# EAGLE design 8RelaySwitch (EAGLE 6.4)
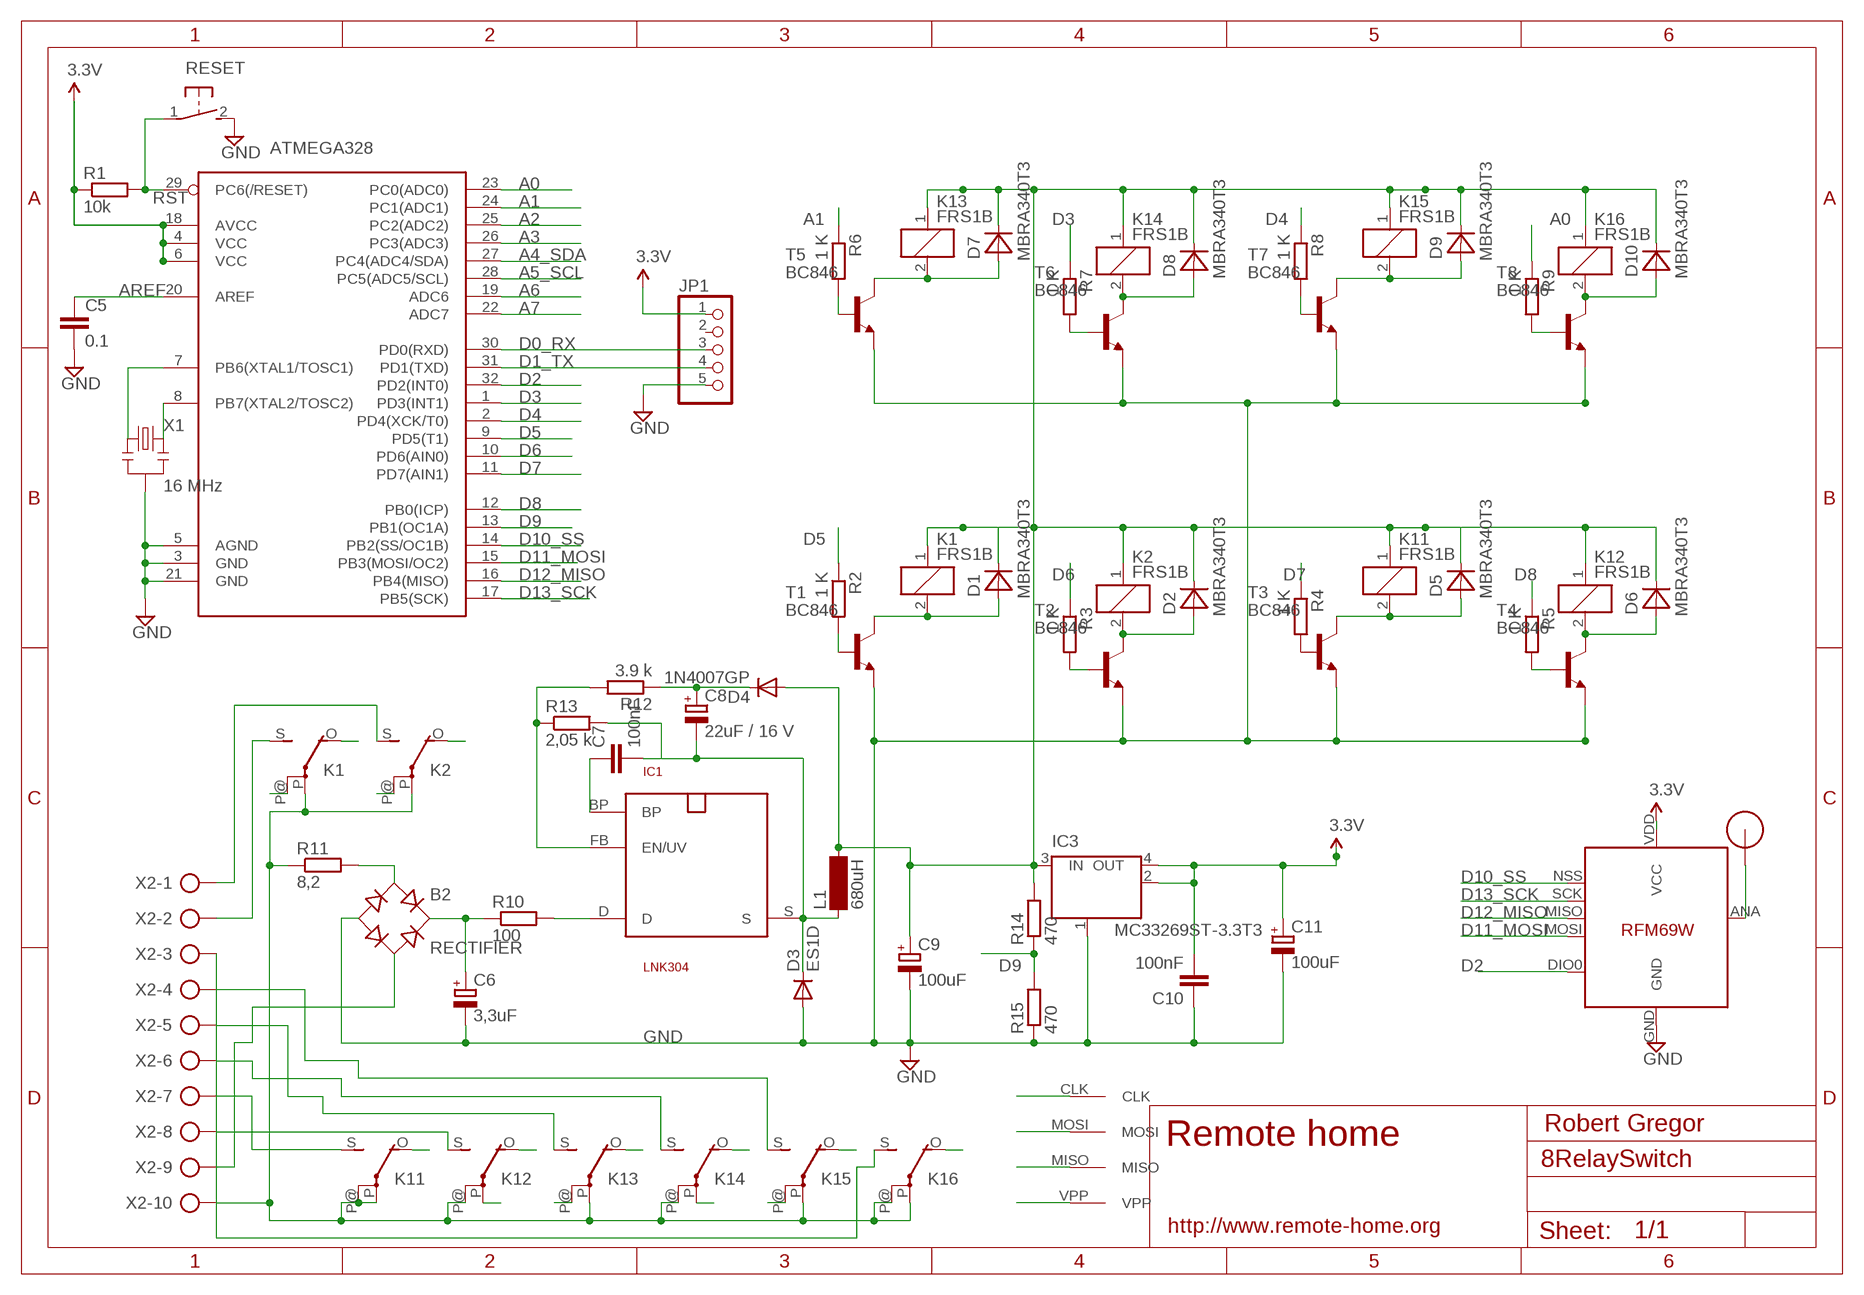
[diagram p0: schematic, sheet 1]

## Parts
ATMEGA328  ATMega-328  ATMEGA168/328TQFP32  [TQFP32-08]
B2  RECTIFIER  RECTIFIER-S40  [TO-269AA]
C5  0.1  C-EUC2012  [C2012]
C6  3,3uF  CPOL-EUE5-10.5  [E5-10,5]
C7  100nF  C-EUC2012  [C2012]
C8  22uF / 16 V  CPOL-EUSMCC  [SMC_C]
C9  100uF  CPOL-EUSMCB  [SMC_B]
C10  100nF  C-EUC2012  [C2012]
C11  100uF  CPOL-EUSMCB  [SMC_B]
D1  MBRA340T3  [SMA]
D2  MBRA340T3  [SMA]
D3  ES1D  DIODE-DO214AC  [DO214AC]
D4  1N4007GP  DIODE-DO214AA  [DO214AA]
D5  MBRA340T3  [SMA]
D6  MBRA340T3  [SMA]
D7  MBRA340T3  [SMA]
D8  MBRA340T3  [SMA]
D9  MBRA340T3  [SMA]
D10  MBRA340T3  [SMA]
IC1  LNK304  SO-8C  [SO-8C]
IC3  MC33269ST-3.3T3  [SOT223]
JP1  PINHD-1X05_2.54-S  [1X05-S]
K1  FRS1B  [FRS1B]
K2  FRS1B  [FRS1B]
K11  FRS1B  [FRS1B]
K12  FRS1B  [FRS1B]
K13  FRS1B  [FRS1B]
K14  FRS1B  [FRS1B]
K15  FRS1B  [FRS1B]
K16  FRS1B  [FRS1B]
L1  680uH  BS11  [BS11]
R1  10k  R-EU_R2012  [R2012]
R2  1 K  R-EU_M2012  [M2012]
R3  1 K  R-EU_M2012  [M2012]
R4  1 K  R-EU_M2012  [M2012]
R5  1 K  R-EU_M2012  [M2012]
R6  1 K  R-EU_M2012  [M2012]
R7  1 K  R-EU_M2012  [M2012]
R8  1 K  R-EU_M2012  [M2012]
R9  1 K  R-EU_M2012  [M2012]
R10  100  R-EU_R2512W  [R2512W]
R11  8,2  R-EU_0411/12  [0411/12]
R12  3.9 k  R-EU_M2012  [M2012]
R13  2,05 k  R-EU_M2012  [M2012]
R14  470  R-EU_M2012  [M2012]
R15  470  R-EU_M2012  [M2012]
RESET  DTSM-3  [DTSM-3]
T1  BC846  [SOT23]
T2  BC846  [SOT23]
T3  BC846  [SOT23]
T4  BC846  [SOT23]
T5  BC846  [SOT23]
T6  BC846  [SOT23]
T7  BC846  [SOT23]
T8  BC846  [SOT23]
U$1  RFM12B_ANTENNA  [RFM12B-ANTENNA]
U$2  AVRHEADERDIP  [AVRHEADER]
U$5  RFM69  [RFM69W-MINPADS]
X1  16 MHz  RESONATORSMD  [RESONATOR-SMD]
X2  AK500/10  [AK500/10]

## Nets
5V1: C9.+ D1.C D2.C D4.A D5.C D6.C D7.C D8.C D9.C D10.C IC3.3(IN) K1.1 K2.1 K11.1 K12.1 K13.1 K14.1 K15.1 K16.1 L1.2 R14.2
A0: ATMEGA328.23(PC0(ADC0)) R9.1
A1: ATMEGA328.24(PC1(ADC1)) R6.1
A2: ATMEGA328.25(PC2(ADC2))
A3: ATMEGA328.26(PC3(ADC3))
A4_SDA: ATMEGA328.27(PC4(ADC4/SDA))
A5_SCL: ATMEGA328.28(PC5(ADC5/SCL))
A6: ATMEGA328.19(ADC6)
A7: ATMEGA328.22(ADC7)
AREF: ATMEGA328.20(AREF) C5.1
D0_RX: ATMEGA328.30(PD0(RXD)) JP1.3
D1_TX: ATMEGA328.31(PD1(TXD)) JP1.4
D2: ATMEGA328.32(PD2(INT0)) U$5.DIO0
D3: ATMEGA328.1(PD3(INT1)) R7.1
D4: ATMEGA328.2(PD4(XCK/T0)) R8.1
D5: ATMEGA328.9(PD5(T1)) R2.1
D6: ATMEGA328.10(PD6(AIN0)) R3.1
D7: ATMEGA328.11(PD7(AIN1)) R4.1
D8: ATMEGA328.12(PB0(ICP)) R5.1
D9: ATMEGA328.13(PB1(OC1A)) R14.1 R15.2
D10_SS: ATMEGA328.14(PB2(SS/OC1B)) U$5.NSS(SEL)
D11_MOSI: ATMEGA328.15(PB3(MOSI/OC2)) U$2.MOSI U$5.MOSI
D12_MISO: ATMEGA328.16(PB4(MISO)) U$2.MISO U$5.MISO
D13_SCK: ATMEGA328.17(PB5(SCK)) U$2.CLK U$5.SCK
GND [power]: ATMEGA328.3(GND) ATMEGA328.5(AGND) ATMEGA328.21(GND) B2.- C5.2 C6.- C9.- C10.1 C11.- D3.A IC3.1(GND/ADJ) JP1.5 R15.1 RESET.2 T1.2(E) T2.2(E) T3.2(E) T4.2(E) T5.2(E) T6.2(E) T7.2(E) T8.2(E) U$5.GND X1.2
N$1: ATMEGA328.7(PB6(XTAL1/TOSC1)) X1.1
N$2: R2.2 T1.1(B)
N$3: U$1.P$1 U$5.ANA(ANT)
N$4: D2.A K2.2 T2.3(C)
N$5: D1.A K1.2 T1.3(C)
N$6: R3.2 T2.1(B)
N$7 [220V]: K1.S(2:S) X2.2
N$8 [220V]: K12.P(2:P)
N$9 [220V]: B2.AC2 X2.9
N$10: C7.2 C8.- D3.C IC1.S L1.1 R13.2
N$11 [220V]: K1.P@(2:P)
N$13 [220V]: IC1.D R10.2
N$14 [220V]: B2.+ C6.+ R10.1
N$15 [220V]: B2.AC1 R11.2
N$16 [220V]: K2.P@(2:P)
N$17 [220V]: K1.O(2:O)
N$18: C7.1 IC1.BP
N$19 [220V]: K2.O(2:O)
N$20: C8.+ D4.C R12.1
N$21: ATMEGA328.8(PB7(XTAL2/TOSC2)) X1.3
N$22: D5.A K11.2 T3.3(C)
N$24: R4.2 T3.1(B)
N$25: D6.A K12.2 T4.3(C)
N$26: R5.2 T4.1(B)
N$27: D7.A K13.2 T5.3(C)
N$28: R6.2 T5.1(B)
N$29: D8.A K14.2 T6.3(C)
N$30: R7.2 T6.1(B)
N$31: D9.A K15.2 T7.3(C)
N$32: R8.2 T7.1(B)
N$33: D10.A K16.2 T8.3(C)
N$34: R9.2 T8.1(B)
N$35 [220V]: K14.P(2:P)
N$36 [220V]: K12.S(2:S) X2.8
N$37 [220V]: K11.S(2:S) X2.7
N$38 [220V]: K13.P@(2:P)
N$40 [220V]: K15.P@(2:P)
N$41 [220V]: K1.P(2:P) K2.P(2:P) K11.P(2:P) K11.P@(2:P) K12.P@(2:P) K13.P(2:P) K14.P@(2:P) K15.P(2:P) K16.P(2:P) K16.P@(2:P) R11.1 X2.10
N$42 [220V]: K11.O(2:O)
N$43 [220V]: K12.O(2:O)
N$44 [220V]: K13.O(2:O)
N$45 [220V]: K14.O(2:O)
N$46 [220V]: K15.O(2:O)
N$47 [220V]: K16.S(2:S) X2.3
N$48 [220V]: K2.S(2:S) X2.1
N$50 [220V]: K13.S(2:S) X2.5
N$51 [220V]: K14.S(2:S) X2.6
N$52 [220V]: K15.S(2:S) X2.4
N$53 [220V]: K16.O(2:O)
RST: ATMEGA328.29(PC6(/RESET)) R1.2 RESET.1 U$2.VPP
VCC: ATMEGA328.4(VCC) ATMEGA328.6(VCC) ATMEGA328.18(AVCC) C10.2 C11.+ IC3.2(OUT) IC3.4(OUT) JP1.1 R1.1 U$5.VDD(VCC) ; supply symbol labelled 3.3V
XXX: IC1.FB(EN/UV) R12.2 R13.1
Unconnected: JP1.2

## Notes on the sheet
- Robert Gregor
- Remote home
- http://www.remote-home.org

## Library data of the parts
ATMEGA328 = LowPowerLab:ATMEGA168/328: Atmel 32-pin 8-bit micro, 16k flash.
B2 = rectifier:RECTIFIER-: Rectifier
C5 C7 C10 = resistor:C-EU: CAPACITOR, European symbol
C6 C8 C9 C11 = resistor:CPOL-EU: POLARIZED CAPACITOR, European symbol
D1 D2 D5-D10 = diode:MBRA340T3: Surface Mount Schottky Power Rectifier
D3 D4 = diode:DIODE-: DIODE
IC1 = powerint:SO-8C: 700V MOSFET für Schaltnetz-Trafos. Pin 3 fehlt. SMD
IC3 = linear:MC33269ST*: Adjustable Output Low Dropout Voltage Regulator 800 mA Source: http://www.onsemi.com/pub/Collateral/MC33269-D.PDF
JP1 = pinhead-2:PINHD-1X05: PIN HEADER
K1 K2 K11-K16 = relay:FRS1B: RELAY 1 x switch, same as V23101-D6-A201, Siemens; OC_FARNELL: unknown; OC_NEWARK: unknown
L1 = inductor-neosid:BS: INDUCTOR; OC_FARNELL: unknown; OC_NEWARK: unknown
R1-R15 = resistor:R-EU_: RESISTOR, European symbol
RESET = switch-tact:DTSM-3
T1-T8 = transistor:BC846: NPN TRANSISTOR
U$1 = LowPowerLab:RFM12B_ANTENNA
U$2 = RemoteHome:AVRHEADER
U$5 = LowPowerLab:RFM69
X1 = SparkFun:RESONATOR: Resonator Small SMD resonator. This is the itty bitty 10/20MHz resonators with built in caps. CSTCE10M0G55 and CSTCE20M0V53. Footprint has been reviewed closely but hasn't been tested yet.
X2 = con-ptr500:AK500/10: CONNECTOR; OC_FARNELL: unknown; OC_NEWARK: unknown

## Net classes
1 power: width 0.381 mm, clearance 0.254 mm
2 220V: width 0.381 mm, clearance 0.508 mm

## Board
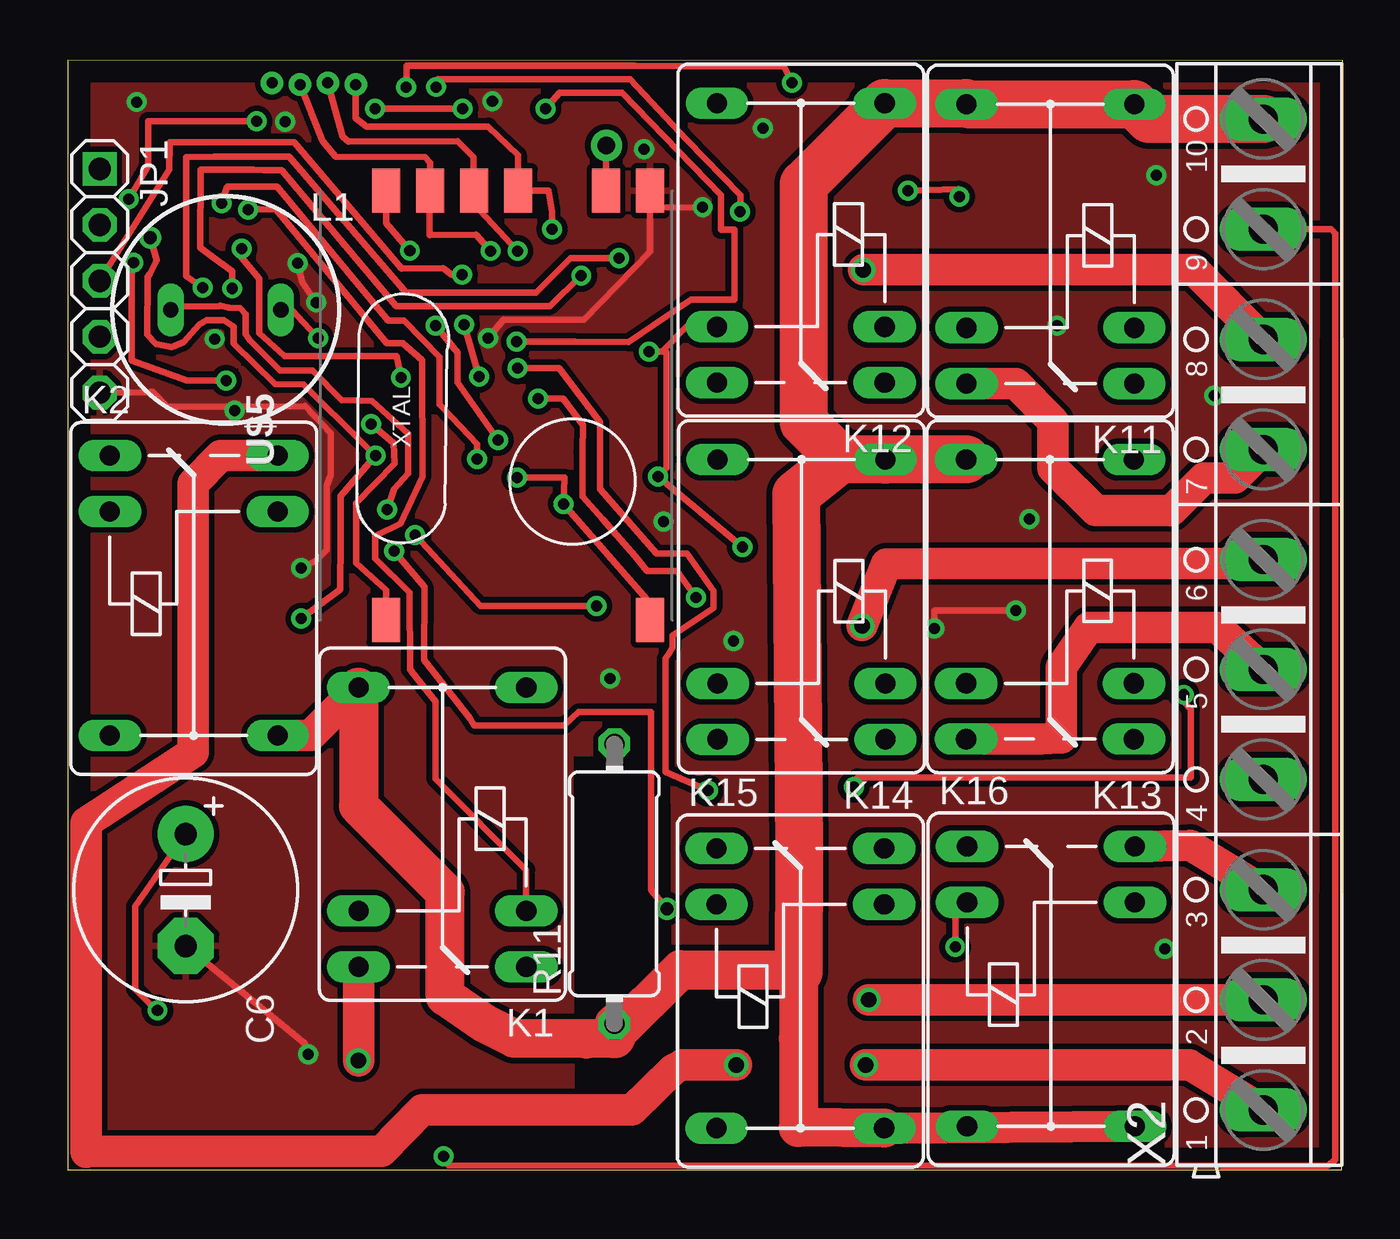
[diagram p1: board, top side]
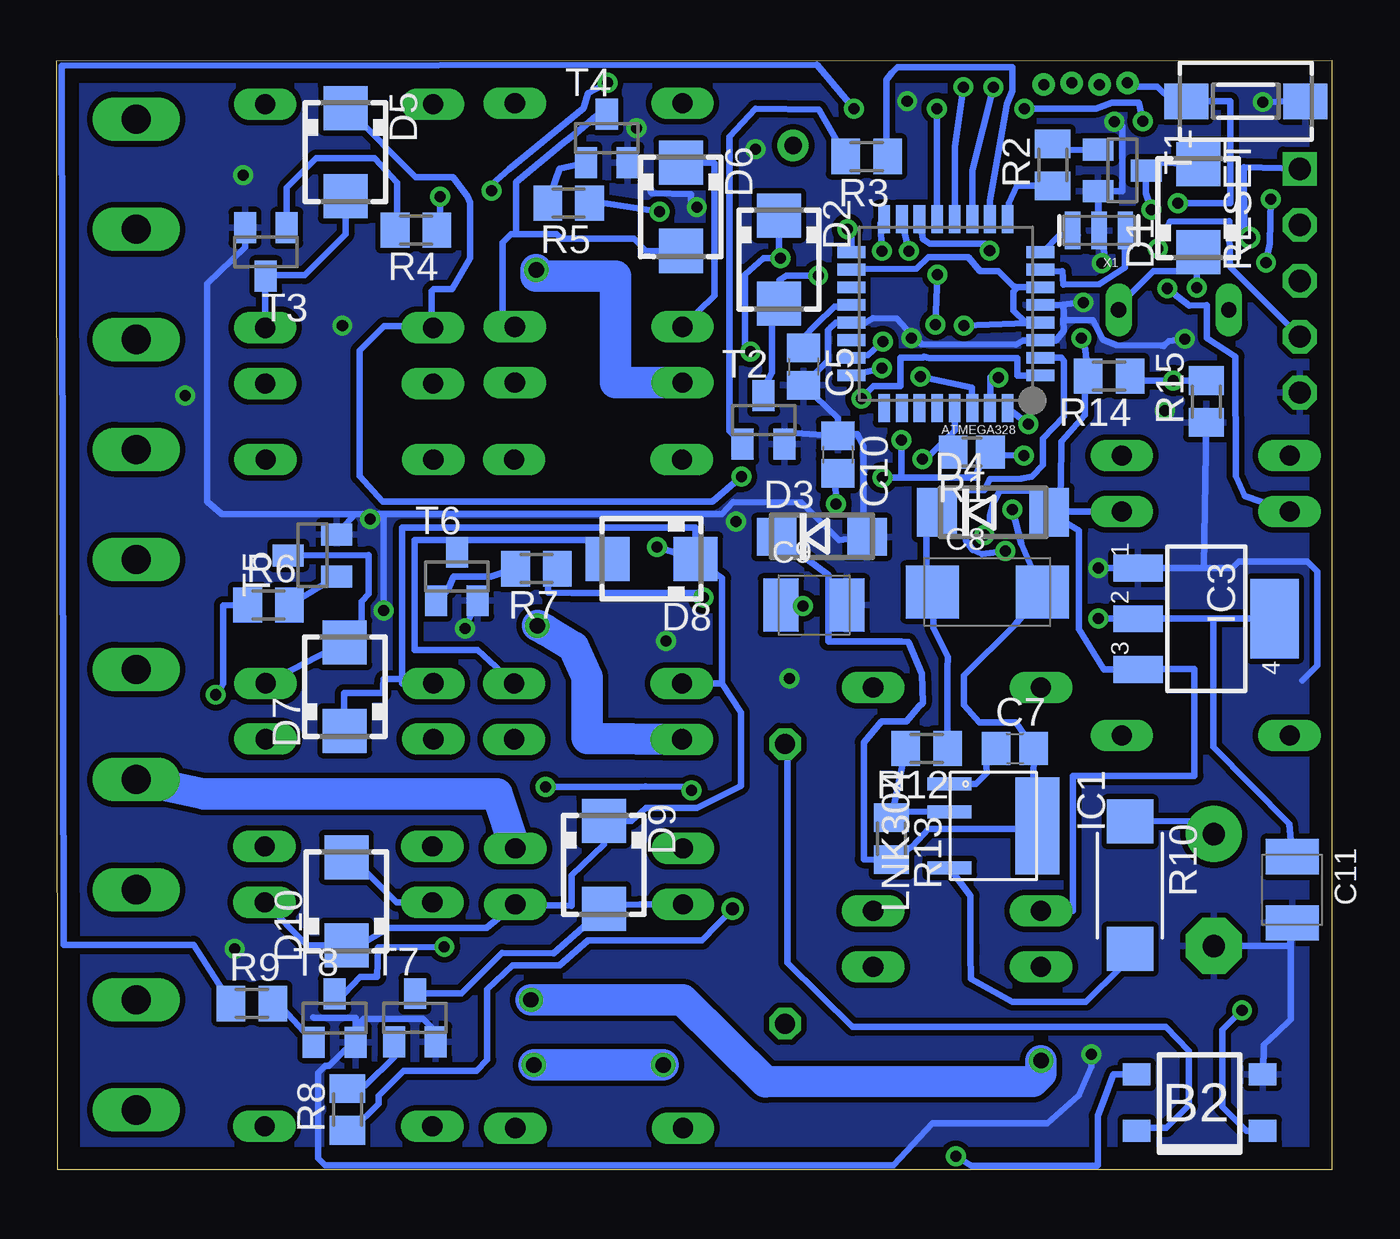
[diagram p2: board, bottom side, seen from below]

Size 57.9 x 50.4 mm. Coordinates in mm from the lower left corner, seen from the top.
Outline: 0,0 57.85,0 57.9,50.38 0,50.4 0,0
Copper layers (1*16): Top 0.035mm / dielectric 1.5mm / Bottom 0.035mm
Design rules "default": minimum track width 10mil, minimum drill 24mil, track to track 8mil, track to pad 8mil, pad to pad 8mil, via to via 8mil, smd to smd 8mil, copper to edge 40mil, drill to drill 8mil, minimum pad ring 10mil, minimum via ring 8mil, stop-mask expansion 4mil, vias tented up to drill 0mil, thermal gap 10mil

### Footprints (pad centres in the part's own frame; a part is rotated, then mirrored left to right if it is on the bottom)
TQFP32-08 = smd 1.27 x 0.533: 1 -4.293,2.8; 2 -4.293,2; 3 -4.293,1.2; 4 -4.293,0.4; 5 -4.293,-0.4; 6 -4.293,-1.2; 7 -4.293,-2; 8 -4.293,-2.8; 17 4.293,-2.8; 18 4.293,-2; 19 4.293,-1.2; 20 4.293,-0.4; 21 4.293,0.4; 22 4.293,1.2; 23 4.293,2; 24 4.293,2.8 | smd 0.533 x 1.27: 9 -2.8,-4.293; 10 -2,-4.293; 11 -1.2,-4.293; 12 -0.4,-4.293; 13 0.4,-4.293; 14 1.2,-4.293; 15 2,-4.293; 16 2.8,-4.293; 25 2.8,4.293; 26 2,4.293; 27 1.2,4.293; 28 0.4,4.293; 29 -0.4,4.293; 30 -1.2,4.293; 31 -2,4.293; 32 -2.8,4.293
TO-269AA = smd 1 x 1.25: + -1.28,-2.855; - 1.28,-2.855; AC1 -1.28,2.855; AC2 1.28,2.855
C2012 = smd 1.3 x 1.5: 1 -0.85,0; 2 0.85,0
E5-10,5 = drill 1.016 pad 2.54: + -2.54,0 | drill 1.016 pad 2.54 octagon: - 2.54,0
SMC_C = smd 2.4 x 2.4: + -2.5,0; - 2.5,0
SMC_B = smd 1.6 x 2.4: + -1.5,0; - 1.5,0
SMA = smd 2 x 2: A 2,0; C -2,0
DO214AC = smd 1.8 x 1.7: A 2.05,0; C -2.05,0
DO214AA = smd 1.8 x 2.2: A 2.55,0; C -2.55,0
SO-8C = smd 0.6 x 2: BP -1.905,-2; D 1.905,-2; FB -0.635,-2 | smd 4.41 x 2: S 0,2
SOT223 = smd 1.219 x 2.235: 1 -2.311,-3.099; 2 0,-3.099; 3 2.311,-3.099 | smd 3.6 x 2.2: 4 0,3.099
1X05-S = drill 1.016 square: 1 -5.08,0 | drill 1.016 octagon: 2 -2.54,0; 3 0,0; 4 2.54,0; 5 5.08,0
FRS1B = drill 0.914 long: 1 0,3.81; 2 0,-3.81; O -2.54,-3.81; P 10.16,3.81; P@ 10.16,-3.81; S -2.54,3.81
BS11 = drill 0.7 long: 1 -2.5,0; 2 2.5,0
R2012 = smd 1.3 x 1.5: 1 -0.85,0; 2 0.85,0
M2012 = smd 1.3 x 1.6: 1 -0.95,0; 2 0.95,0
R2512W = smd 2 x 2.1: 1 -2.896,0; 2 2.896,0
0411/12 = drill 0.914 octagon: 1 -6.35,0; 2 6.35,0
DTSM-3 = smd 2 x 1.6: 1 -2.7,0; 2 2.7,0
SOT23 = smd 1 x 1.4: 1 -0.95,-1.1; 2 0.95,-1.1; 3 0,1.1
RFM12B-ANTENNA = drill 0.8 pad 1.422: P$1 0,0
AVRHEADER = drill 0.5: CLK 2.54,0; MISO 1.27,0.07; MOSI 0,0; VPP -1.27,0.072
RFM69W-MINPADS = smd 2 x 1.27: ANA 8,-5; DIO0 -11.5,5; GND 8,-7; MISO 8,1; MOSI 8,3; NSS 8,5; SCK 8,-1; VDD -11.5,-7
RESONATOR-SMD = smd 0.7 x 1.7: 1 -1.2,0; 2 0,0; 3 1.2,0
AK500/10 = drill 1.321 long: 1 -22.504,0; 2 -17.501,0; 3 -12.497,0; 4 -7.493,0; 5 -2.489,0; 6 2.489,0; 7 7.493,0; 8 12.497,0; 9 17.501,0; 10 22.504,0

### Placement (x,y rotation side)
ATMEGA328  17.52,38.88 180 bottom
B2  5.99,3.05 90 bottom
C5  23.99,36.48 270 bottom
C6  5.35,12.7 270 top
C7  14.38,19.13 0 bottom
C8  15.64,26.24 0 bottom
C9  23.51,25.65 0 bottom
C10  22.43,32.48 270 bottom
C11  1.79,12.72 270 bottom
D1  6.06,43.68 90 bottom
D2  25.1,41.34 270 bottom
D3  23.15,28.75 0 bottom
D4  15.38,29.86 0 bottom
D5  44.79,46.22 270 bottom
D6  29.55,43.73 270 bottom
D7  44.82,21.94 90 bottom
D8  30.89,27.75 180 bottom
D9  33.05,13.85 270 bottom
D10  44.74,12.19 90 bottom
IC1  15.35,15.62 270 bottom
IC3  5.69,25.03 270 bottom
JP1  1.44,40.38 270 top
K1  17.01,11.75 90 top
K2  5.71,29.89 270 top
K11  44.62,38.24 90 top
K12  33.29,38.28 90 top
K13  44.61,22.1 90 top
K14  33.32,22.09 90 top
K15  33.27,12.05 270 top
K16  44.65,12.14 270 top
L1  7.17,39.05 0 top
R1  16.34,32.59 180 bottom
R2  12.67,45.64 90 bottom
R3  21.12,46.02 180 bottom
R4  41.58,42.68 180 bottom
R5  34.65,43.91 180 bottom
R6  48.28,25.65 0 bottom
R7  36.11,27.3 180 bottom
R8  44.69,2.74 90 bottom
R9  49.03,7.55 0 bottom
R10  9.16,12.92 270 bottom
R11  24.82,12.98 90 top
R12  18.39,19.14 180 bottom
R13  19.98,15.03 270 bottom
R14  10.11,36.05 180 bottom
R15  5.69,34.89 90 bottom
RESET  3.9,48.52 0 bottom
T1  9.51,45.39 270 bottom
T2  25.8,34.05 0 bottom
T3  48.4,41.69 180 bottom
T4  32.92,46.84 0 bottom
T5  46.28,27.9 90 bottom
T6  39.73,26.94 0 bottom
T7  41.63,6.9 0 bottom
T8  45.28,6.89 0 bottom
U$1  24.46,46.52 0 top
U$2  10.54,49.29 0 top
U$5  19.45,36.46 90 top
X1  10.57,42.66 180 bottom
X2  54.29,25.22 90 top

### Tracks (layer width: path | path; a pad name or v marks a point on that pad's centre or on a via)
5V1  (via drill 0.5)
  Top 0.305: v11.36,37.77 11.24,37.9 10.19,39.05 L1.2 | v24.01,25.61 22.24,25.61 18.75,25.61 v15.78,28.84 | v25.03,41.4 24.08,41.4 23.14,41.41 22.82,41.41 21.27,39.84 15.35,39.84 10.06,46.02 6.65,46.02 5.36,46 5.37,40.58 v6.12,40.06 | K12.1 28.1,38.28 26.98,37.17 v26.39,37.17 27.17,37.17 27.2,37.14 27.2,31.88 27.18,31.86 26.83,31.53 v26.8,31.49 v30.64,28.28
  Bottom 0.305: D4.A 11.47,29.04 11.47,24.56 10.34,22.72 IC3.3 8.79,22.74 6.23,22.74 6.23,17.89 11.75,17.89 11.75,11.75 K1.1 | 12.9,29.89 D4.A | v11.36,37.77 11.19,37.24 R14.2 11.21,36.2 11.2,34.28 12.28,33.08 12.3,31.16 12.37,30.24 | 12.37,30.24 12.39,29.88 D4.A | C9.+ v24.01,25.61 | v15.78,28.84 15.52,28.71 15.5,29.04 15.52,29.7 15.35,30.28 15.06,30.85 12.37,30.84 12.37,30.24 | D4.A | v6.12,40.06 6.12,40.87 | L1.2 9.67,39.25 8.1,40.82 6.17,40.82 6.12,40.87 | v26.39,37.17 26.65,37.5 26.65,40.66 25.79,41.4 v25.03,41.4 25.1,41.8 D2.C | D6.C 28.02,45.72 28.02,43.31 28.02,39.7 K12.1 | D5.C 44.68,48.17 41.6,45.09 39.91,45.09 39.24,44.2 39.13,43.92 39.13,42.47 39.13,41.4 39.94,40 40.79,40 40.88,39.91 40.88,38.31 K11.1 40.89,38.32 43.03,38.32 44.14,37.2 44.14,31.51 43.1,30.35 33.1,30.36 33.1,30.35 28.12,30.35 v26.8,31.49 | D1.C 6.06,40.93 6.12,40.87 | K2.1 12.79,29.89 D4.A | 27.68,22.09 27.68,26.87 28.89,27.72 D8.C | K13.1 42.2,22.1 42.2,22.29 | 42.2,22.29 42.2,29.17 28.89,29.17 D8.C | D7.C 44.85,21.65 43.1,21.65 43.05,22.29 42.2,22.29 | K16.1 46.52,10.19 D10.C 44.17,10.19 42.8,10.98 38.37,10.98 K15.1 37.02,12 34.95,12 34.51,11.99 34.51,13.37 33.05,14.78 33.05,14.96 D9.C 31.8,15.85 31.12,16.43 28.82,16.43 26.83,17.44 26.83,20.78 27.68,22.09 | K14.1 27.68,22.09 | v30.64,28.28 D8.C
A0  (via drill 0.5)
  Top 0.305: v20.39,37.6 23.02,37.6 25.45,37.59 28.3,39.52 30.27,39.52 30.27,42.69 29.65,42.69 29.67,44.26 25.16,48.92 22.32,48.92 v21.7,48.19
  Bottom 0.305: ATMEGA328.23 21.07,37 v20.39,37.6 | v21.7,48.19 23.37,50.2 57.67,50.15 57.57,10.22 51.68,10.22 R9.1
A1  (via drill 0.5)
  Top 0.305: v20.42,36.4 22.3,36.41 24.18,33.96 24.17,30.92 26.73,27.98 28.11,27.98 29.31,26.28 29.32,25.52 27.45,24.28 27.45,23.72 27.3,23.45 27.15,23.21 27.14,19.15 27.14,18.08 v29.06,17.22 | v35.69,17.39 35.85,17.83 51,17.83 51,20.91 50.67,21.25 v50.67,21.58
  Bottom 0.305: ATMEGA328.24 v20.42,36.4 | v29.06,17.22 29.4,17.4 31.15,17.4 31.47,17.38 35.12,17.38 v35.69,17.39 | R6.1 50.34,25.64 50.34,22.09 50.6,21.54 v50.67,21.58
AREF
  Bottom 0.305: C5.1 24,37.33 24.01,37.34 24.01,37.78 23.41,38.38 | 23.41,38.38 | 23.41,38.38 22.58,39.21 21.88,39.21 ATMEGA328.20
D0_RX  (via drill 0.5)
  Top 0.305: v17.91,40.65 17.43,40.65 17.04,40.94 15.16,40.92 10.29,46.66 4.61,46.68 4.59,45.43 JP1.3 | v17.98,38.39 v18.66,36.02
  Bottom 0.305: v17.91,40.65 v17.98,38.39 | v18.66,36.02 16.34,35.52 ATMEGA328.30
D1_TX  (via drill 0.5)
  Top 0.305: v7.88,41.83 7.88,41.43 8.69,40.47 8.69,38 9.85,36.95 14.94,36.95 v15.12,35.98
  Bottom 0.305: v7.88,41.83 7.34,43.07 4.64,43.09 4.62,41.06 4.57,40.98 JP1.4 | v15.12,35.98 15.5,36 15.51,35.56 15.51,34.6 ATMEGA328.31
D2  (via drill 0.5)
  Top 0.305: U$5.DIO0 14.45,26.34 13.1,27.56 13.1,30.29 14.84,32.07 14.8,33 v13.78,33.86
  Bottom 0.305: v13.78,33.86 14.71,34.58 ATMEGA328.32
D3  (via drill 0.5)
  Top 0.305: v21.36,35.02 22.48,35.02 23.39,33.83 23.37,32.61 23.38,30.57 24.27,29.57 25.75,27.89 26.3,27.2 27.66,27.19 v28.52,25.98
  Bottom 0.305: ATMEGA328.1 14.28,36.08 14.27,36.87 18.27,36.87 18.51,36.92 18.57,36.88 19.58,36.89 19.57,35.59 20.02,35.59 20.8,35.59 v21.36,35.02 | v28.52,25.98 28.71,26.2 30.77,26.19 34.42,26.19 34.49,26.19 35.57,26.22 35.57,27.26 R7.1
D4  (via drill 0.5, 0.6)
  Top 0.305: v14.81,28.1 16.2,26.47 16.19,23.15 18.26,20.49 18.45,20.19 22.54,20.19 23.2,20.79 26.48,20.79 26.49,12.7 v27.21,11.85
  Bottom 0.305: R8.1 44.49,1.79 43.29,3 43.29,3.35 42.14,4.5 38.83,4.5 38.35,4.99 38.35,8.2 37.19,9.29 35.07,9.29 33.77,10.41 28.59,10.41 v27.21,11.85 | ATMEGA328.2 12.27,36.88 12.16,36.72 12.16,34.21 13.11,33.2 13.11,32 13.62,31.49 14.09,31.4 15.53,31.37 15.77,30.87 16.6,30.86 16.62,28.58 16.29,28.15 15.89,27.96 v14.81,28.1
D5
  Bottom 0.305: R2.1 13.88,44.7 14.29,44.7 14.66,43.89 ATMEGA328.9
D6
  Bottom 0.305: ATMEGA328.10 15.52,44.02 14.75,48.39 14.49,49.01 14.49,50.09 17.53,50.09 19.72,50.09 19.97,49.83 20.21,49.51 20.21,47.09 R3.1
D7  (via drill 0.5)
  Top 0.305: v15.35,49.17 15.38,49.35 15.38,50.14 20.41,50.14 21.87,50.15 25.76,50.15 27.76,50.13 32.53,50.13 v32.88,49.37 | v38.15,44.48 40.46,44.53 v40.48,44.19
  Bottom 0.305: ATMEGA328.11 16.32,45.4 v15.35,49.17 | v32.88,49.37 33.77,48.88 33.97,48.22 37.36,45.44 38.13,44.77 v38.15,44.48 | v40.48,44.19 40.48,43.2 R4.1
D8  (via drill 0.5)
  Top 0.305: v16.72,49.18 16.75,49.33 16.8,49.52 25.52,49.52 28.11,46.76 30.55,44.26 v30.52,43.51
  Bottom 0.305: ATMEGA328.12 17.12,46.47 v16.72,49.18 | v30.52,43.51 33.18,43.93 R5.1
D9  (via drill 0.5)
  Top 0.305: v7.18,35.84 5.41,35.84 2.89,36.74 2.89,40.62 v2.98,41.19 | v2.77,44.08 3.64,45.58 3.64,47.63 v8.57,47.63 | v17.92,48.2 v13.95,48.2
  Bottom 0.305: 8.8,35.84 R14.1 8.88,35.83 v7.18,35.84 R15.2 | v2.98,41.19 2.8,42.07 v2.77,44.08 | ATMEGA328.13 v17.92,48.2 | v13.95,48.2 10.71,48.2 9.98,48.47 8.75,48.47 v8.57,47.63
D10_SS  (via drill 0.5)
  Top 0.305: U$5.NSS 14.45,42.98 v15.53,41.74
  Bottom 0.305: v15.53,41.74 15.71,42.07 17.07,42.05 18.25,42.05 18.55,42.27 18.7,43.16 ATMEGA328.14
D11_MOSI  (via drill 0.5)
  Top 0.305: v19.2,41.73 18.55,42.46 16.42,42.45 U$5.MOSI 16.46,44.48 16.46,45.73 16.23,46 12.17,46.01 11.57,46.71 U$2.MOSI
  Bottom 0.305: v19.2,41.73 19.54,43.15 ATMEGA328.15
D12_MISO  (via drill 0.5)
  Top 0.305: v20.42,41.73 18.45,43.85 U$5.MISO 18.43,44.48 18.43,46 17.7,46.71 12.74,46.69 12.49,46.92 U$2.MISO
  Bottom 0.305: v20.42,41.73 20.49,43 ATMEGA328.16
D13_SCK  (via drill 0.5)
  Top 0.305: v21.98,42.72 21.98,43.51 21.82,44.47 U$5.SCK 20.44,46.09 19.08,47.38 13.57,47.38 13.08,47.76 U$2.CLK
  Bottom 0.305: ATMEGA328.17 21.81,42.84 v21.98,42.72
GND  (via drill 0.5)
  Top 0.305: U$5.GND 26.45,43.89 | 26.45,43.89 26.45,41.71 23.44,38.61 19.8,38.61 v19.08,37.78 | v10.59,27.32 11.28,27.67 11.75,28.14 11.75,31.06 11.93,31.56 11.93,33.45 10.78,34.7 8.7,34.67 8.69,34.67 4.52,34.67 3.86,35.32 3.75,35.32 JP1.5 | v10.44,41.18 10.63,40.32 v11.27,39.4 | v28.83,43.72 26.52,43.71 26.45,43.89 | v39.35,24.59 39.35,25.4 v43.06,25.4 | v10.92,5.25 10.76,5.75 C6.-
  Bottom 0.305: 5.74,27.34 IC3.1 10.39,27.34 v10.59,27.32 | 5.74,27.34 4.5,27.34 4.22,27.62 1.1,27.62 0.65,27.16 0.65,22.9 1.33,22.22 | 10.58,44.26 X1.2 10.33,41.65 v10.44,41.18 | C10.1 22.43,34.15 C5.2 22.87,36.75 22.87,38.13 22.52,38.48 ATMEGA328.21 21.16,38.48 20.84,38.68 19.74,38.66 18.9,37.72 18.63,37.51 14.34,37.49 13.99,37.66 13.24,37.66 ATMEGA328.3 13.21,37.66 12.53,37.66 12.15,38.11 12.18,38.59 | C10.1 24.35,33.45 | C10.1 22.43,33.44 22.39,33.41 21.53,33.41 21.26,32.85 21.26,29 D3.A 22.37,28.6 24.07,30.3 27.2,30.33 27.68,29.79 27.77,29.77 43.05,29.77 | ATMEGA328.5 12.45,39.28 12.17,39.3 | 12.17,39.3 12.15,38.87 12.18,38.59 | 7.62,37.44 9.77,37.45 10.39,37.71 10.85,38.59 12.18,38.59 | v11.27,39.4 11.68,39.35 12.17,39.3 | T4.2 32.09,45.6 31.06,44.89 30.89,44.36 29.1,44.32 29.1,43.86 v28.83,43.72 | T3.2 49.35,41.9 51.07,40.26 51.07,30.36 50.4,29.77 44.35,29.77 | 44.35,29.77 43.05,29.77 | T6.2 v39.35,24.59 | v43.06,25.4 43.05,29.77 | T5.2 44.35,29.77 | B2.- 3.09,4.94 3.07,5.17 3.07,5.68 2.48,6.23 1.86,6.84 1.86,10.22 C11.- 1.89,10.17 C6.- | T7.2 40.68,6.28 41.26,6.86 43.96,6.86 | 43.96,6.86 44.33,6.49 | 44.33,6.49 T8.2 | 43.96,6.86 43.97,6.86 43.97,6.27 45.52,4.71 45.7,4.71 46.02,4.39 46.02,0.53 45.7,0.21 19.89,0.21 18.14,2.11 12.9,2.11 11.49,3.38 10.92,4.68 v10.92,5.25 | RESET.2 1.78,48.52 v3.12,48.5 | v9.86,47.6 9.5,47.39 9.5,44.45 T1.2 | R15.1 5.79,27.39 5.74,27.34 | v6.67,37.74 7.39,37.65 7.62,37.43 | 7.62,37.43 7.62,37.41 | 7.62,37.43 7.62,37.44 7.6,37.46 | 7.6,37.46 | 7.6,37.46 7.63,37.43 7.74,37.43 | 44.33,6.49 44.33,6.89 46.21,6.89 46.26,6.92
  other vias: 49.43,45.18 44.93,38.34 52.06,35.16 49.82,10.03 19.28,48.53 26.17,46.35 24.62,22.32 7.56,34.49 43.68,29.56 31.56,47.31 27.05,29.43 30.22,24.03
  pour Top: 27,50.17 0.15,50.23 0.2,46.62 0.2,0.22 22.88,0.2 22.83,18.91 27.44,18.97 27.51,18.97 27.6,0.19 57.68,0.19 57.73,50.13 32.49,50.19
  pour Bottom: 25.19,50.18 0.2,50.21 0.2,0.2 57.67,0.2 57.76,42.84 57.76,50.19
N$1
  Bottom 0.305: ATMEGA328.7 13.22,40.84 13.18,40.79 12.23,40.82 12.18,40.19 10.54,40.21 9.38,40.96 9.38,42.19 X1.1
N$2
  Bottom 0.305: R2.2 12.3,46.31 T1.1
N$3
  Top 0.305: U$5.ANA 24.45,46.06 U$1.P$1
N$4  (via drill 0.5)
  Top 0.305: v7.47,40.03 7.45,40.81 6.65,41.41 6,41.89 6.02,45.42 8.43,45.41 8.88,45.41 9.71,45.41 14.91,39.23 15.71,39.23 15.86,39.23 16.37,39.22 16.7,39.23 19.62,39.22 19.73,39.23 21.89,39.23 v23.32,40.6
  Bottom 0.305: T2.3 25.8,35.51 25.41,36.2 25.41,38.67 25.75,39.33 D2.A 25.09,39.35 25.09,40.41 24.75,40.6 v23.32,40.6 | K2.2 3.95,30.59 4.35,31.51 4.36,36.94 5.66,37.77 5.66,38 5.66,39.28 6.45,39.25 v7.47,40.03
N$5  (via drill 0.5)
  Top 0.305: K1.2 20.82,13.63 16.69,17.76 16.69,21.28 16.12,22 15.54,22.73 15.51,26.21 13.95,27.75 13.96,28.78 15.1,29.35 16.1,31.48 16.08,36.77 15.21,37.55 14.47,37.54 9.45,43.62 8.68,43.63 v8.2,43.61
  Bottom 0.305: v8.2,43.61 8.45,44.35 T1.3 7.73,45.73 D1.A
N$6
  Bottom 0.305: R3.2 23.29,48.16 26.16,48.18 27.34,46.91 27.34,44.28 27.34,33.54 T2.1
N$7  (via drill 0.7)
  Top 1.422: X2.2 v36.36,7.72 | v13.19,4.96 K1.S
  Bottom 1.422: v36.36,7.72 29.48,7.72 25.71,4 13.56,4.02 13.19,4.39 v13.19,4.96
N$9  (via drill 0.5)
  Top 0.305: X2.9 57.37,42.72 57.57,42.52 57.57,0.45 57.23,0.19 52.41,0.19 17.28,0.2 17.07,0.41 v17.07,0.62
  Bottom 0.305: B2.AC2 9.9,4.33 10.31,3.23 10.62,2.44 10.62,0.21 10.65,0.18 16.36,0.18 v17.07,0.62
N$10  (via drill 0.5)
  Top 0.305: L1.1 4.9,39.28 5.12,39.21 6.86,39.23 6.91,39.25 7.29,39.17 7.82,39.13 8.07,38.86 8.08,37.96 8.26,37.69 9.63,36.3 11.12,36.31 12.43,34.96 13.81,34.91 15.46,33.43 15.46,31.62 14.8,30.92 v14.5,29.99
  Bottom 0.305: v14.5,29.99 14.08,28.41 C8.- 14.39,24.74 16.69,22.44 16.69,21.11 16,20.32 14.33,20.32 C7.2 13.56,15.83 IC1.S 13.48,15.49 18.3,15.49 19.03,14.68 R13.2 20,14.07 21.24,14.1 21.24,19.41 20.91,19.82 20.43,20.36 19.3,20.36 18.74,21.05 18.57,21.19 18.6,22.51 19.22,23.98 19.53,23.99 21.05,23.99 22.86,23.99 22.86,25.64 22.86,27.01 D3.C
N$13
  Bottom 0.305: R10.2 9.58,9.19 11.15,7.64 14.49,7.64 16.39,8.67 16.39,9.84 16.4,10.16 16.39,12.45 IC1.D
N$14  (via drill 0.5)
  Top 0.305: v4.07,7.24 4,7.24 3.05,8.2 3.05,11.95 C6.+
  Bottom 0.305: R10.1 6.3,15.84 C6.+ | B2.+ 3.87,1.77 4.96,2.86 4.96,6.35 v4.07,7.24
N$15
  Bottom 0.305: B2.AC1 8.85,1.83 8.77,1.91 7.5,1.91 6.48,2.92 6.48,5.4 7.52,6.49 21.75,6.49 24.72,9.4 24.72,19.23 R11.2
N$18
  Bottom 0.305: C7.1 15.74,19.14 15.66,18.02 16.16,17.52 IC1.BP
N$20
  Bottom 0.305: R12.1 17.44,22.77 17.43,23.29 18.08,24.6 C8.+ 18.35,26.09 18.41,26.59 18.41,29.11 D4.C
N$21
  Bottom 0.305: ATMEGA328.8 13.11,41.68 12.35,42.44 11.53,42.44 X1.3
N$22
  Bottom 0.305: K11.2 48.43,40.56 T3.3 48.36,40.63 46.65,40.63 44.79,42.49 D5.A
N$24
  Bottom 0.305: T3.1 47.45,44.6 46.11,45.94 43.47,45.94 42.45,44.82 42.45,43.18 R4.2
N$25
  Bottom 0.305: D6.A 31.13,41.73 31.67,42.28 34.98,42.28 35.2,42.5 36.77,42.5 | 36.77,42.5 37.26,42.5 37.66,42.1 37.66,38.85 K12.2 | T4.3 33.4,47.86 34.31,47.08 34.88,46.64 37.03,44.85 37.03,42.5 36.77,42.5
N$26
  Bottom 0.305: R5.2 35.06,45.48 T4.1
N$27
  Bottom 0.305: T5.3 43.74,27.92 43.74,26.16 44.05,25.81 44.05,23.69 D7.A K13.2
N$28
  Bottom 0.305: T5.1 R6.2
N$29
  Bottom 0.305: D8.A 33.38,27.33 33.74,27.33 33.74,28.6 40.16,28.6 | 40.16,28.6 41.65,28.6 41.65,23.61 38.8,23.61 K14.2 | T6.3 40.08,28.52 40.16,28.6
N$30
  Bottom 0.305: T6.1 41.03,25.39 40.14,26.3 | 40.14,26.3 | 40.14,26.3 39.88,26.95 38.18,26.95 R7.2
N$31
  Bottom 0.305: K15.2 31.42,12.04 33.07,12.03 D9.A 35.34,9.84 37.66,9.86 39.52,8.02 T7.3
N$32
  Bottom 0.305: T7.1 42.58,5.12 43.86,3.84 44.55,3.84 R8.2
N$33  (via drill 0.5)
  Top 0.305: v40.3,10.13 40.3,11.59 K16.2
  Bottom 0.305: K16.2 42.46,12.14 44.08,13.76 44.31,13.76 D10.A | v40.3,10.13 43.31,10.11 43.34,8.76 44.11,8.76 44.85,7.99 T8.3
N$34
  Bottom 0.305: R9.2 47.84,7.55 T8.1
N$36  (via drill 0.7)
  Top 1.422: v36.13,40.87 51.13,40.87 X2.8
  Bottom 1.422: K12.S 32.51,35.74 32.51,40.59 36.13,40.59 v36.13,40.87
N$37
  Top 1.422: K11.S 43.06,35.7 44.74,34.01 44.74,31.88 46.69,29.93 50.11,29.93 51.6,31.42 53,31.42 X2.7
N$41
  Top 0.305: K16.P@ K15.P
  Top 1.422: K2.P 11.02,19.73 K1.P | K16.P K15.P | 24.86,5.97 24.86,6.14 | 33.09,9.09 33.18,9
  Top 1.778: K1.P 13.2,16.54 17.13,12.6 17.13,7.87 18.91,6.66 20.25,5.97 23.54,5.94 24.77,5.97 R11.1 24.91,6.06 24.86,5.97 | 33.18,9 33.17,5.96 33.18,1.92 K15.P | 24.86,6.14 27.8,9.09 33.09,9.09
  Top 2.184: X2.10 49.11,47.72 K11.P@ K11.P 40.77,48.44 K12.P@ 33.42,44.77 33.42,33.94 35.1,32.26 | K13.P K14.P@ | K13.P 35.1,32.26 | K13.P 35.1,32.26 | 35.1,32.26 35.08,32.29 | 35.08,32.29 | 35.08,32.29 33.07,30.68 33.2,14.47 33.18,9
N$47
  Top 1.422: X2.3 50.97,14.73 K16.S
N$48  (via drill 0.7)
  Top 1.422: K2.S 6.93,32.43 5.68,31.18 5.68,18.95 0.84,15.77 0.84,0.79 0.88,0.84 14.25,0.84 16.1,2.73 25.63,2.73 27.49,4.54 27.89,4.76 v30.36,4.76 | X2.1 50.92,4.76 v36.23,4.76
  Bottom 1.422: v36.23,4.76 v30.36,4.76
N$50
  Top 1.422: K13.S 44.19,19.56 45.12,19.61 45.12,22.83 46.34,24.6 46.37,24.64 52.2,24.64 X2.5
N$51  (via drill 0.7)
  Top 1.422: v36.07,24.71 37.16,27.52 38.91,27.54 54.12,27.54 X2.6
  Bottom 1.422: K14.S 33.78,19.59 33.83,19.63 33.83,22.38 34.44,23.73 35.69,24.5 v36.07,24.71
N$52
  Bottom 1.422: X2.4 51.23,17.07 37.9,17.07 K15.S
RST  (via drill 0.5)
  Top 0.305: v18.59,32.28 18.59,32.96 17.44,34.17 16.88,34.76 16.88,35.14 16.88,36.91 15.27,38.56 14.55,38.56 9.5,44.64 7.23,44.64 v6.99,43.9
  Bottom 0.305: 17.12,33.57 ATMEGA328.29 17.12,33.57 | 17.12,33.57 17.42,33.27 17.42,32.51 R1.2 | U$2.VPP 9.2,49.19 7.91,49.19 7.24,48.52 RESET.1 4.6,48.54 4.6,43.9 v6.99,43.9 | 17.12,33.57 18.32,32.37 18.62,32.37 v18.59,32.28
VCC  (via drill 0.5, 0.6)
  Top 0.305: v10.6,25.03 12.37,26.36 12.38,28.65 12.38,30.6 v13.97,32.45 13.43,32.95 10.71,35.66 9.41,35.67 7.53,37.53 7.53,38.28 7.07,38.59 6.31,38.6 5.96,38.39 5.25,37.59 4.7,37.36 4.02,37.49 3.59,37.94 3.62,40.56 3.7,40.67 4.03,41.31 v3.73,42.34 | U$5.VDD 26.44,25.75 v22.52,30.25 22.55,31.44 v20.4,31.44 | v16.7,38.34 17.69,37.1 17.7,35.76 v19.54,33.14
  Bottom 0.305: IC3.4 5.32,25.03 | 5.32,25.03 IC3.2 9.51,25.03 v10.6,25.03 | ATMEGA328.6 14.26,40.08 | 14.26,40.08 14.45,40.12 15.12,40.82 15.97,40.82 16.49,41.46 18.3,41.46 18.32,41.44 18.34,41.44 18.85,40.93 21.79,40.9 ATMEGA328.18 | 14.26,40.08 14.45,39.89 14.45,39.03 13.89,38.48 ATMEGA328.4 v16.7,38.34 | v13.97,32.45 15.75,32.48 R1.1 15.82,32.47 16.19,31.44 18.64,31.44 19.53,31.44 | v22.52,30.25 22.53,31.39 C10.2 | 19.53,31.44 v20.4,31.44 | JP1.1 3.98,45.54 3.97,42.67 v3.73,42.34 | v19.54,33.14 19.54,31.45 19.53,31.44 | C11.+ 1.93,15.71 5.38,19.21 5.38,24.97 5.32,25.03
XXX
  Bottom 0.305: IC1.FB 18.18,16.25 19.44,16.28 19.69,16.28 R13.1 20,16 R12.2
